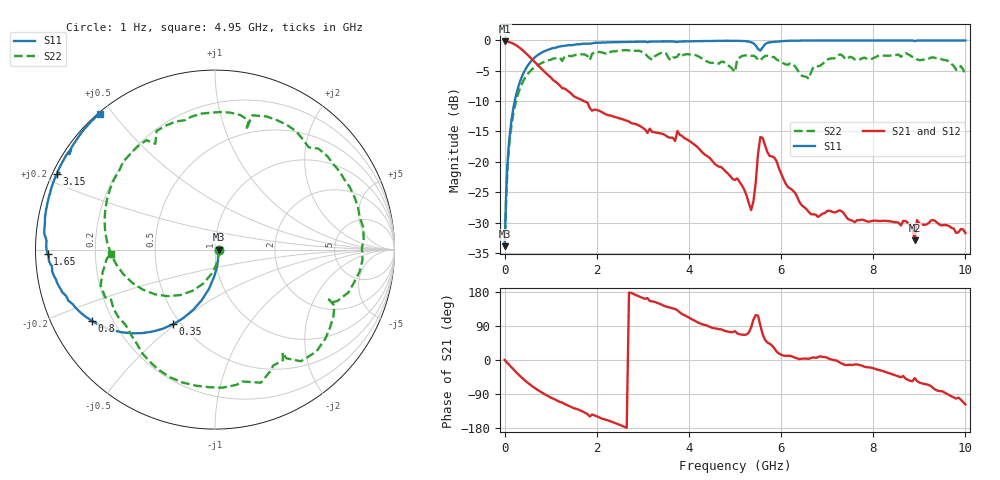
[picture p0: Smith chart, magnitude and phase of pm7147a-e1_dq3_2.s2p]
# GHz S DB R 50
! S-Parameters data
! Freq  dbS11  angS11  dbS21  angS21  dbS12  angS12  dbS22  angS22
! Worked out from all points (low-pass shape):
!   279 points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, 1 Hz to 10 GHz, reference 50 ohm
!   highest |S21| = -0.18 dB at 7.9 Hz (marker M1); lowest = -32.9 dB at 8.9 GHz (marker M2)
!   |S21| within 3 dB of the highest: start of sweep to 603.2 MHz
!   lowest |S11| = -33.9 dB at 631 Hz (marker M3), VSWR 1.04, Z = 52.1 - j7.52e-05 ohm
!   |S11| at or under -10 dB: start of sweep to 219.8 MHz
!   |S22| runs from -33.9 to -1.6 dB; largest |S21 - S12| = 0
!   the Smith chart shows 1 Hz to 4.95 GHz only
!   S11 on the Smith chart (normalised r, x): 1 Hz: 1.04, -0.00; 350 MHz: 0.46, -0.49; 800 MHz: 0.12, -0.27; 1.65 GHz: 0.03, -0.01; 3.15 GHz: 0.01, +0.23; 4.95 GHz: 0.00, +0.46
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1e-09  -33.89 -0.0  -0.18 -0.0  -0.18 -0.0  -33.89 -0.0
7.9e-09  -33.89 -0.0  -0.18 -0.0  -0.18 -0.0  -33.89 -0.0
6.31e-07  -33.89 -0.0  -0.18 -0.0  -0.18 -0.0  -33.89 -0.0
0.1  -16.43 -91.8  -0.28 -13.2  -0.28 -13.2  -17.28 -98.2
0.35  -6.45 -119.2  -1.35 -44.0  -1.35 -44.0  -7.57 -143.5
0.8  -2.02 -149.9  -4.69 -85.3  -4.69 -85.3  -3.74 160.2
1.65  -0.60 -178.6  -9.71 -133.6  -9.71 -133.6  -2.30 87.7
1.7  -0.55 -179.9  -9.92 -136.5  -9.92 -136.5  -2.29 83.6
2.6  -0.26 162.5  -13.10 -176.4  -13.10 -176.4  -1.61 20.7
3.15  -0.22 154.4  -14.53 155.9  -14.53 155.9  -2.94 -24.4
3.35  -0.17 151.1  -15.26 149.0  -15.26 149.0  -2.22 -34.2
4.05  -0.14 142.0  -16.77 108.4  -16.77 108.4  -2.32 -97.9
4.95  -0.06 130.2  -22.84 73.4  -22.84 73.4  -4.76 -177.8
5.05  -0.07 128.8  -22.73 70.0  -22.73 70.0  -3.01 -176.8
5.35  -0.30 122.9  -27.94 85.9  -27.94 85.9  -2.52 149.8
5.6  -1.17 129.8  -16.05 67.9  -16.05 67.9  -2.87 132.8
6.3  -0.04 119.3  -25.07 6.2  -25.07 6.2  -4.25 80.2
6.7  -0.02 115.1  -28.65 7.0  -28.65 7.0  -4.38 83.1
8.35  -0.01 101.0  -29.79 -34.8  -29.79 -34.8  -2.52 -1.4
8.9  -0.12 96.1  -32.95 -47.8  -32.95 -47.8  -2.80 -37.7
9.45  -0.01 93.4  -30.39 -82.1  -30.39 -82.1  -2.99 -76.3
10  -0.01 89.9  -31.73 -117.2  -31.73 -117.2  -5.64 -122.3
